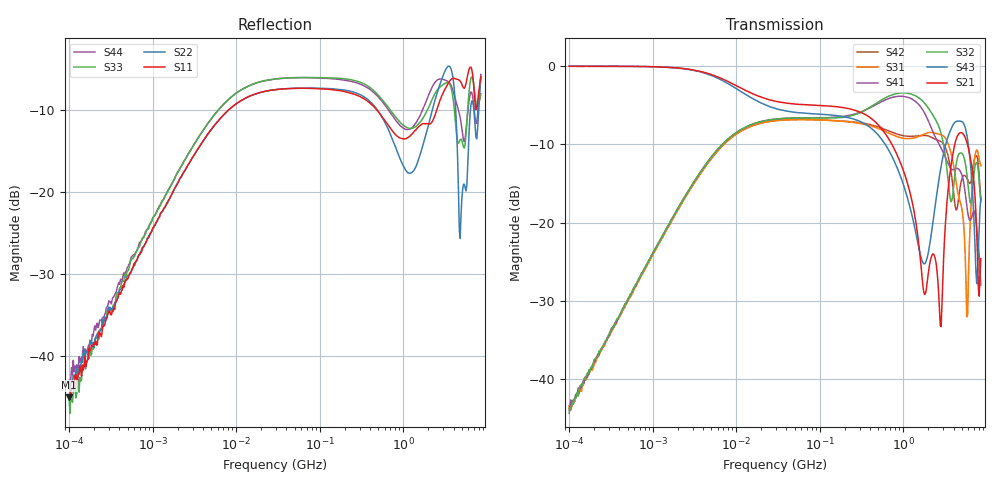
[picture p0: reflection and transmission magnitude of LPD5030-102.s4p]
# MHz S MA R 50
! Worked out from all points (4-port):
!   498 points, 100 kHz to 8.5 GHz, reference 50 ohm
!   strongest paths, dB at 100 kHz, 1.698 MHz, 29.49 MHz, 500.7 MHz, 8.5 GHz:
!     S21: 0.0, -0.2, -4.5, -7.5, -24.6
!     S43: 0.0, -0.2, -5.4, -8.8, -16.9
!     S32: -44.3, -19.5, -6.8, -4.6, -17.3
!     S41: -43.9, -19.5, -6.8, -4.8, -28.0
!     S31: -43.7, -19.7, -7.0, -8.0, -12.7
!     S42: -43.4, -19.7, -7.0, -7.8, -17.1
!   lowest |S11| = -45.0 dB at 100 kHz (marker M1), VSWR 1.01, Z = 50 + j0.557 ohm
!   |S11| at or under -10 dB: start of sweep to 8.057 MHz; 485.7 MHz to 2.507 GHz (2.021 GHz wide, 135 % of centre)
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0.1  0.005594 94.4  0.9945 -0.3  0.006637 -90.6  0.006298 89.4
     0.9947 -0.4  0.006797 90.9  0.006785 84.6  0.006317 -93.8
     0.006545 -89.6  0.006082 90.1  0.005592 92.6  0.9949 -0.4
     0.006373 87.0  0.006773 -96.7  0.9959 -0.4  0.007117 105.3
17.44001  0.3997 20.2  0.6491 -18.1  0.4238 -161.5  0.433 21.3
          0.6491 -18.1  0.3993 20.2  0.4333 21.3  0.4234 -161.6
          0.4234 -161.5  0.4333 21.3  0.4646 20.5  0.6004 -22.0
          0.4328 21.3  0.4234 -161.6  0.6002 -22.0  0.4647 20.4
407.6417  0.3471 -70.5  0.465 -90.9  0.4144 75.0  0.5436 -46.7
          0.4648 -90.9  0.355 -77.2  0.5483 -43.1  0.4217 73.0
          0.4141 74.9  0.5487 -43.1  0.4324 -71.0  0.4025 -96.5
          0.5438 -46.7  0.4214 73.0  0.4025 -96.4  0.4211 -70.0
1248.181  0.2239 -162.5  0.1435 124.1  0.3444 -91.6  0.6173 175.1
          0.1439 124.1  0.1316 -163.6  0.6607 -178.5  0.3554 -97.7
          0.3446 -91.6  0.6606 -178.5  0.2448 -169.8  0.1163 96.8
          0.6172 175.1  0.3552 -97.7  0.1163 97.0  0.2458 -161.5
2776.003  0.3672 36.5  0.02261 33.3  0.365 11.7  0.307 -44.4
          0.02207 33.9  0.4618 26.3  0.3864 -50.3  0.3312 8.9
          0.365 11.7  0.3863 -50.3  0.4402 15.2  0.2136 120.2
          0.3072 -44.4  0.3311 8.9  0.2136 120.3  0.4907 6.8
4484.409  0.4877 -176.1  0.3591 -175.4  0.157 101.9  0.2214 102.3
          0.3596 -175.2  0.1561 129.9  0.2622 134.2  0.1287 150.5
          0.1573 101.8  0.2624 134.3  0.2006 175.5  0.4442 -173.4
          0.2217 102.0  0.1292 150.7  0.4444 -173.4  0.3284 170.2
8500  0.5067 -33.4  0.05927 75.9  0.2294 1.2  0.03897 161.6
      0.05902 76.1  0.5038 -19.3  0.1349 -64.5  0.1423 -53.1
      0.2306 1.1  0.1362 -64.6  0.3997 -27.5  0.1437 54.6
      0.03999 160.8  0.1402 -52.8  0.1436 54.5  0.5239 -25.3
